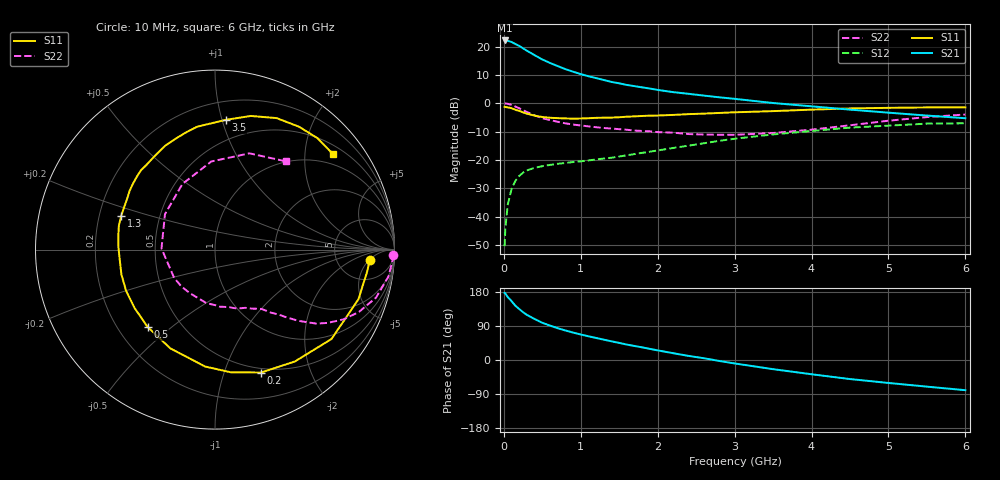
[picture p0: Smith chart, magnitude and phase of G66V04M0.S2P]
! SIEMENS Small Signal Semiconductors
! BFG193
! Si NPN RF Bipolar Junction Transistor in SOT223
! VCE = 6 V  IC = 4 mA
! Common Emitter S-Parameters:  August  1996
# GHz  S  MA  R  50
!  f  S11  S21  S12  S22
! GHz  MAG  ANG  MAG  ANG  MAG  ANG  MAG  ANG
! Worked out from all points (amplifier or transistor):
!   36 points, 10 MHz to 6 GHz, reference 50 ohm
!   highest |S21| = 22.2 dB at 10 MHz (marker M1)
!   |S21| within 3 dB of that: start of sweep to 263.3 MHz
!   unconditionally stable (mu >= 1): 1.217 GHz to 2.514 GHz
!   at 250 MHz: K = 0.28, MSG = 21.9 dB, |S12| = -24.5 dB
!   at 1.4 GHz: K = 1.09, MAG = 11.6 dB, |S12| = -19.2 dB
!   at 6 GHz: K = 0.88, MSG = 0.9 dB, |S12| = -7.1 dB
!   S11 on the Smith chart (normalised r, x): 10 MHz: 11, -5; 200 MHz: 0.46, -1.34; 500 MHz: 0.32, -0.42; 1.3 GHz: 0.29, +0.16; 3.5 GHz: 0.34, +1.03; 6 GHz: 0.71, +2.66
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0.01  0.8634 -3.8  12.82 177.1  0.003 91.6  0.993 -1.7
0.02  0.8573 -7.9  12.8 175.4  0.0063 89.2  0.9907 -3.6
0.05  0.8457 -19.1  12.68 166.2  0.0159 79.9  0.9782 -8.8
0.1  0.8182 -37.5  12.04 155.5  0.0307 71.4  0.9363 -16.6
0.15  0.766 -54.4  11.12 143.2  0.0426 62.3  0.8743 -23.4
0.2  0.7316 -69.4  10.26 134.5  0.052 56.5  0.8148 -28.5
0.25  0.6891 -82.7  9.317 126.1  0.0596 51.0  0.7495 -33.0
0.3  0.6539 -94.8  8.452 119.1  0.0652 47.3  0.7002 -36.1
0.4  0.604 -114.3  7.046 108.1  0.0724 41.5  0.6093 -40.6
0.5  0.5716 -131.0  5.923 98.2  0.0774 37.6  0.5455 -43.6
0.6  0.5538 -143.9  5.143 90.8  0.0816 35.8  0.5034 -45.8
0.7  0.546 -155.2  4.525 84.0  0.0852 34.7  0.4708 -48.3
0.9  0.5337 -173.5  3.603 72.4  0.0916 34.2  0.4206 -51.9
1.1  0.5439 172.3  2.996 62.6  0.0979 35.0  0.3907 -57.4
1.3  0.5553 160.4  2.567 53.7  0.1058 36.0  0.3654 -62.6
1.6  0.5785 145.1  2.101 40.6  0.1206 36.6  0.3402 -72.9
2.2  0.6218 122.2  1.571 18.0  0.1623 34.6  0.3025 -98.8
2.8  0.6737 103.6  1.273 -2.5  0.2168 27.2  0.2774 -132.9
3.5  0.7256 85.2  1.009 -24.2  0.2815 12.9  0.2981 178.8
4.5  0.8091 64.9  0.771 -50.3  0.3714 -8.4  0.4083 116.4
5.5  0.8433 47.5  0.606 -70.3  0.4364 -35.4  0.5696 70.3
6  0.8459 39.0  0.544 -79.7  0.4428 -50.5  0.6321 51.0
